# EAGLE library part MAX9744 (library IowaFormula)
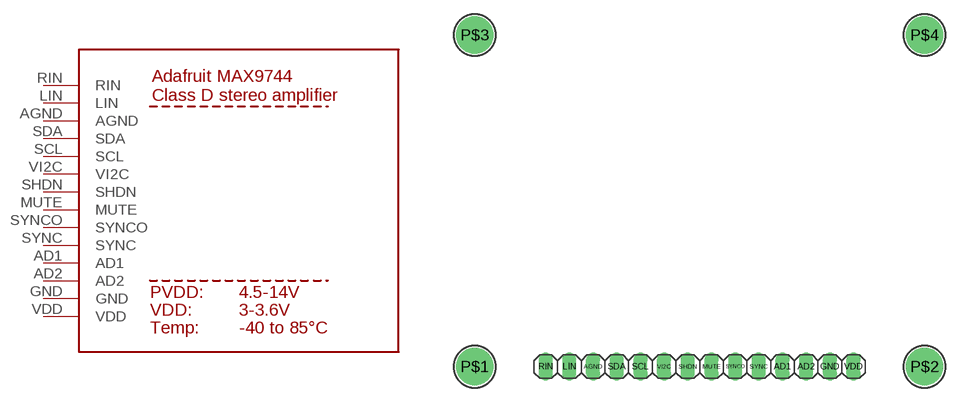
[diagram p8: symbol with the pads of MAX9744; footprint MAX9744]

Designator prefix -

## MAX9744  [MAX9744]
AD1  AD1
AD2  AD2
AGND  AGND
GND  GND
LIN  LIN
MUTE  MUTE
RIN  RIN
SCL  SCL
SDA  SDA
SHDN  SHDN
SYNC  SYNC
SYNCO  SYNCO
VDD  VDD
VI2C  VI2C

## Footprint MAX9744 (pad centres in mm)
drill 1.016 long: AD1 33.02,0; AD2 35.56,0; AGND 12.7,0; GND 38.1,0; LIN 10.16,0; MUTE 25.4,0; RIN 7.62,0; SCL 17.78,0; SDA 15.24,0; SHDN 22.86,0; SYNC 30.48,0; SYNCO 27.94,0; VDD 40.64,0; VI2C 20.32,0
drill 2.5 pad 4: P$1 0,0; P$2 48.26,0; P$3 0,35.56; P$4 48.26,35.56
